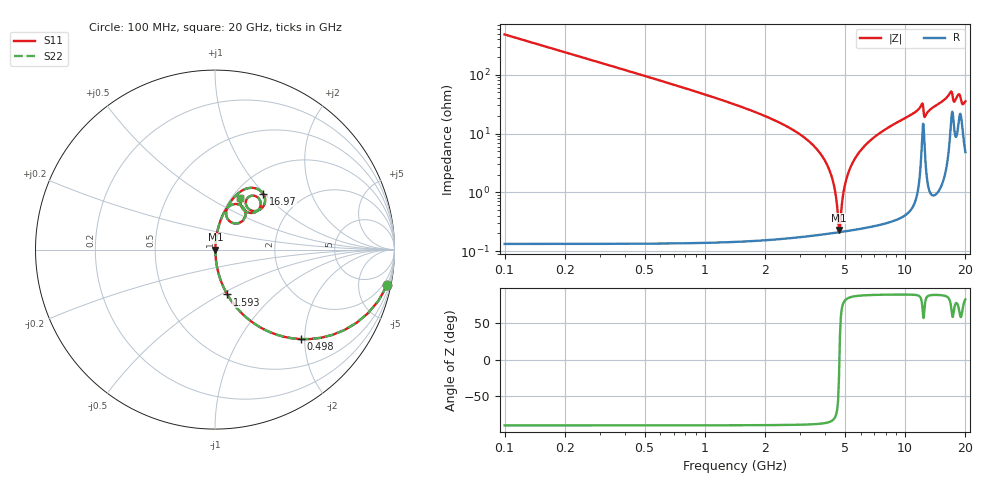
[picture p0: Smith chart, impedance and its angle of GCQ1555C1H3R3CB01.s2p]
!Murata Part Number: GCQ1555C1H3R3CB01
!These Parameters are Measured in Series Mode Connection
!Data Generated on Mar 13, 2026
!  o--ll--o
!Port1  Port2
!  o------o
!Operation Temp=25[degC], DC Bias Voltage=0[V]
!Freq. Start=100[MHz] Stop=20[GHz] 401[Steps]
# Hz S RI R 50
!Freq.(Hz) S11(Real) S11(Imag) S21(Real) S21(Imag) S12(Real) S12(Imag) S22(Real) S22(Imag)
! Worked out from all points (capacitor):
!   401 points, 100 MHz to 20 GHz, reference 50 ohm
!   read as one part in series: C = 3.3 pF near 199.5 MHz
!   lowest |Z| = 228 mohm at 4.677 GHz (marker M1)
!   series resonance near 4.697 GHz, so ESL is about 350 pH
!   S11 on the Smith chart (normalised r, x): 100 MHz: 1.00, -9.64; 498 MHz: 1.00, -1.92; 1.593 GHz: 1.00, -0.54; 16.97 GHz: 1.31, +0.99; 20 GHz: 1.10, +0.70
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1e8  0.9587 -0.1989  0.0413 0.1989  0.0413 0.1989  0.9587 -0.1989
4.98e8  0.4784 -0.4988  0.5216 0.4988  0.5216 0.4988  0.4784 -0.4988
9.4575e8  0.1939 -0.394  0.8061 0.394  0.8061 0.394  0.1939 -0.394
1.5925e9  0.0683 -0.2495  0.9317 0.2495  0.9317 0.2495  0.0683 -0.2495
3.43325e9  0.0061 -0.0652  0.9939 0.0652  0.9939 0.0652  0.0061 -0.0652
4.22925e9  0.00247 -0.0216  0.9975 0.0216  0.9975 0.0216  0.00247 -0.0216
4.42825e9  0.00219 -0.0122  0.9978 0.0122  0.9978 0.0122  0.00219 -0.0122
4.677e9  0.0021 -0.000895  0.9979 0.000895  0.9979 0.000895  0.0021 -0.000895
4.7765e9  0.00213 0.00345  0.9979 -0.00345  0.9979 -0.00345  0.00213 0.00345
5.02525e9  0.00237 0.0139  0.9976 -0.0139  0.9976 -0.0139  0.00237 0.0139
5.32375e9  0.00291 0.0259  0.9971 -0.0259  0.9971 -0.0259  0.00291 0.0259
6.7665e9  0.00864 0.0775  0.9914 -0.0775  0.9914 -0.0775  0.00864 0.0775
1.005e10  0.0367 0.1772  0.9633 -0.1772  0.9633 -0.1772  0.0367 0.1772
1.208975e10  0.1255 0.2533  0.8745 -0.2533  0.8745 -0.2533  0.1255 0.2533
1.25375e10  0.0782 0.1608  0.9218 -0.1608  0.9218 -0.1608  0.0782 0.1608
1.338325e10  0.0701 0.2373  0.9299 -0.2373  0.9299 -0.2373  0.0701 0.2373
1.67165e10  0.2244 0.3418  0.7756 -0.3418  0.7756 -0.3418  0.2244 0.3418
1.696525e10  0.2681 0.3118  0.7319 -0.3118  0.7319 -0.3118  0.2681 0.3118
1.75125e10  0.1872 0.227  0.8128 -0.227  0.8128 -0.227  0.1872 0.227
1.845775e10  0.2372 0.2914  0.7628 -0.2914  0.7628 -0.2914  0.2372 0.2914
1.925375e10  0.1756 0.2103  0.8244 -0.2103  0.8244 -0.2103  0.1756 0.2103
2e10  0.1417 0.2864  0.8583 -0.2864  0.8583 -0.2864  0.1417 0.2864
